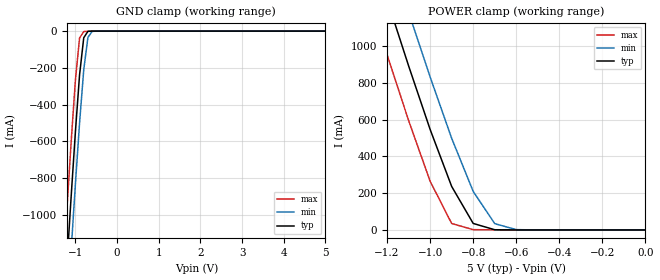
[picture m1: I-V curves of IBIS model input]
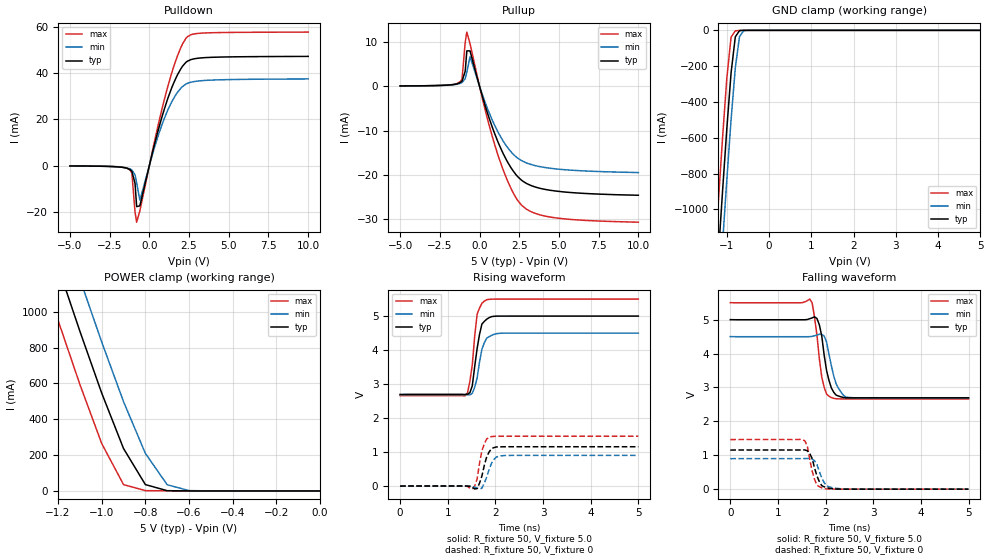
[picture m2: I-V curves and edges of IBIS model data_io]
| SOJ package &  Industrial operation.
[IBIS Ver]   3.2
[Comment Char]   |_char
[File name]   as7c1025b_soji.ibs
[File Rev]   1.0
[Date]   May 26, 2004 10:18:24 AM
[Source]
Alliance Semiconductor Corporation
[Notes]
This model  is for SOJ package & Industrial operation.
[Disclaimer]
Data is for modeling purpose only and is not guaranted.
This IBIS model is provided on an "AS IS" basis and Alliance Semiconductor makes
absolutely no warranty with respect to the information contained
herein.The entire risk as to quality and performance
is with the Customer. ACCORDINGLY, IN NO EVENT SHALL THE COMPANY BE
LIABLE FOR ANY DAMAGES, WHETHER IN CONTRACT OR TORT,INCLUDING ANY
LOST PROFITS OR OTHER INCIDENTAL, CONSEQUENTIAL, EXEMPLARY, OR
PUNITIVE DAMAGES ARISING OUT OF THE USE OR APPLICATION OF THE IBIS
model provided in this package.
[Copyright]
Alliance Semiconductor Corporation
| soj  Package & Industrial operation.
[Component]   AS7C1025B_SOJI
Si_location Pin
Timing_location Pin
[Manufacturer]   Alliance Semiconductor Corporation
[Package]
R_pkg   400.6m   286.6m   514.6m
L_pkg   8.541nH   5.418nH   11.663nH
C_pkg   1.870pF   1.203pF   2.538pF
[Pin] signal_name   model_name
1   A0   input
2   A1   input
3   A2   input
4   A3   input
5   NCE   input
6   IO0   data_io
7   IO1   data_io
8   VCC   POWER
9   GND   GND
10   IO2   data_io
11   IO3   data_io
12   NWE   input
13   A4   input
14   A5   input
15   A6   input
16   A7   input
17   A8   input
18   A9   input
19   A10   input
20   A11   input
21   A12   input
22   IO4   data_io
23   IO5   data_io
24   VCC   POWER
25   GND   GND
26   IO6   data_io
27   IO7   data_io
28   NOE   input
29   A13   input
30   A14   input
31   A15   input
32   A16   input
| Models and submodels in the file (2): input (Input), data_io (I/O)
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[Model]   input
Model_type Input
Vinh=2.2V
Vinl=0.8V
C_comp   4pF   4pF   4pF
[Model Spec]
[Temperature Range] 25   85   -40
[Voltage Range]   5.0   4.5   5.5
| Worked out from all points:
|   GND clamp passes 1 mA (typ) near -0.67 V on its own axis
|   POWER clamp passes 1 mA (typ) near -0.68 V on its own axis
[GND Clamp]
-5V       -16.01A    -16.28A    -15.75A
-1.3V     -1.622A    -1.916A    -1.322A
-1.2V     -1.253A    -1.547A    -953.4mA
-1.1V     -892.6mA   -1.184A    -596mA
-1V       -547.3mA   -832.1mA   -266.1mA
-900mV    -237.4mA   -499.3mA   -37.66mA
-800mV    -36.26mA   -209.9mA   -2.709mA
-700mV    -1.383mA   -34.75mA   -458.6uA
-600mV    -81.45uA   -1.835mA   -48.66uA
5V        292.5pA    86.47uA    -195.3pA
[POWER Clamp]
-5V       16.01A     16.27A     15.75A
-1.3V     1.621A     1.915A     1.322A
-1.2V     1.252A     1.546A     952.5mA
-1.1V     891.7mA    1.183A     594.7mA
-1V       546.1mA    831.3mA    264.7mA
-900mV    236.6mA    498.2mA    35.19mA
-800mV    35.4mA     209.4mA    1.73mA
-700mV    1.248mA    34.46mA    445.9uA
-600mV    85.03uA    1.813mA    86.82uA
0V        292.5pA    2.095nA    135pA
[Model]   data_io
Model_type I/O
Enable Active-High
Polarity Non-Inverting
Vinh=2.2V
Vinl=0.8V
Vref=1.728V
Vmeas=1.5V
Rref=168
Cref=30pF
C_comp   4pF   4pF   4pF
[Temperature Range] 25   85   -40
[Voltage Range]   5.0   4.5   5.5
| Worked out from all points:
|   slope of the pulldown table from 0 to 0.75 V, typ, clamps not added: 37.5 ohm
|   slope of the pullup table from 0 to 0.75 V, typ, clamps not added: 86.3 ohm
|   GND clamp passes 1 mA (typ) near -0.67 V on its own axis
|   POWER clamp passes 1 mA (typ) near -0.68 V on its own axis
|   falling waveform, R_fixture 50, V_fixture 5.0: 20-80 % time 166ps typ, 194ps min, 152ps max; typ from 5 V to 2.7 V
|   falling waveform, R_fixture 50, V_fixture 0: 20-80 % time 154ps typ, 156ps min, 138ps max; typ from 1.16 V to 0.002 V
|   rising waveform, R_fixture 50, V_fixture 5.0: 20-80 % time 146ps typ, 154ps min, 127ps max; typ from 2.69 V to 5 V
|   rising waveform, R_fixture 50, V_fixture 0: 20-80 % time 139ps typ, 149ps min, 124ps max; typ from 0 V to 1.16 V
[Pullup]
-5V       80uA       70uA       70uA
-1.2V     863uA      669uA      1.092mA
-1.1V     1.172mA    848uA      1.674mA
-900mV    3.44mA     1.737mA    9.973mA
-800mV    8.002mA    3.2mA      12.24mA
-600mV    8.001mA    6.666mA    9.641mA
300mV     -3.74mA    -3.123mA   -4.556mA
1.1V      -12.04mA   -9.899mA   -14.87mA
1.8V      -17.34mA   -14.01mA   -21.67mA
2.6V      -21.1mA    -16.71mA   -26.69mA
4.5V      -23.53mA   -18.55mA   -29.59mA
10V       -24.63mA   -19.51mA   -30.72mA
[Pulldown]
-5V       -150uA     -150uA     -120uA
-1.2V     -1.84mA    -1.479mA   -2.07mA
-1.1V     -2.529mA   -1.917mA   -3.263mA
-900mV    -7.724mA   -4.021mA   -20.18mA
-800mV    -17.8mA    -7.454mA   -24.55mA
-600mV    -17.46mA   -14.98mA   -19.72mA
300mV     8.509mA    7.287mA    9.717mA
1.1V      27.83mA    23.1mA     32.73mA
1.7V      38.37mA    31.04mA    46.23mA
2.3V      44.76mA    35.33mA    55.17mA
3.5V      46.82mA    36.93mA    57.52mA
10V       47.36mA    37.58mA    57.9mA
[GND Clamp]
-5V       -16.01A    -16.28A    -15.75A
-1.3V     -1.622A    -1.916A    -1.322A
-1.2V     -1.253A    -1.547A    -953.4mA
-1.1V     -892.6mA   -1.184A    -596mA
-1V       -547.3mA   -832.1mA   -266.1mA
-900mV    -237.4mA   -499.3mA   -37.66mA
-800mV    -36.26mA   -209.9mA   -2.709mA
-700mV    -1.383mA   -34.75mA   -458.6uA
-600mV    -81.45uA   -1.835mA   -48.66uA
5V        292.5pA    86.47uA    -195.3pA
[POWER Clamp]
-5V       16.01A     16.27A     15.75A
-1.3V     1.621A     1.915A     1.322A
-1.2V     1.252A     1.546A     952.5mA
-1.1V     891.7mA    1.183A     594.7mA
-1V       546.1mA    831.3mA    264.7mA
-900mV    236.6mA    498.2mA    35.19mA
-800mV    35.4mA     209.4mA    1.73mA
-700mV    1.248mA    34.46mA    445.9uA
-600mV    85.03uA    1.813mA    86.82uA
0V        292.5pA    2.095nA    135pA
[Falling Waveform]
R_fixture=50
V_fixture=5.0
V_fixture_min=4.5
V_fixture_max=5.5
0s        5V         4.5V       5.5V
1.667ns   5.026V     4.498V     5.606V
1.717ns   5.052V     4.506V     5.495V
1.768ns   5.082V     4.525V     5.07V
1.869ns   4.848V     4.57V      3.851V
1.97ns    3.957V     4.516V     3.009V
2.121ns   2.985V     3.641V     2.7V
2.222ns   2.773V     3.103V     2.667V
2.424ns   2.694V     2.719V     2.66V
5ns       2.696V     2.688V     2.66V
[Falling Waveform]
R_fixture=50
V_fixture=0
V_fixture_min=0
V_fixture_max=0
0s        1.155V     900.6mV    1.463V
1.566ns   1.159V     904.6mV    1.426V
1.616ns   1.134V     905.8mV    1.277V
1.667ns   1.055V     906.1mV    885.3mV
1.768ns   630.4mV    839.3mV    294mV
1.869ns   223.9mV    521.6mV    75.75mV
1.97ns    72.37mV    195.8mV    22.68mV
2.121ns   19.64mV    53.83mV    4.69mV
2.424ns   2.522mV    5.993mV    2.531mV
5ns       2.452mV    2.397mV    2.491mV
[Rising Waveform]
R_fixture=50
V_fixture=5.0
V_fixture_min=4.5
V_fixture_max=5.5
0s        2.694V     2.687V     2.658V
1.364ns   2.691V     2.687V     2.652V
1.414ns   2.701V     2.685V     2.741V
1.515ns   2.949V     2.729V     3.573V
1.566ns   3.52V      2.906V     4.421V
1.616ns   4.042V     3.178V     5.055V
1.717ns   4.764V     4.026V     5.372V
1.818ns   4.906V     4.348V     5.479V
2.121ns   4.996V     4.493V     5.496V
5ns       4.996V     4.497V     5.496V
[Rising Waveform]
R_fixture=50
V_fixture=0
V_fixture_min=0
V_fixture_max=0
0s        0V         647.5nV    0V
1.364ns   3.513mV    2.818mV    3.909mV
1.515ns   -32.3mV    -5.34mV    -77.13mV
1.616ns   -70.03mV   -59.72mV   206mV
1.717ns   298.9mV    -58.02mV   1.045V
1.818ns   866.3mV    269.8mV    1.389V
1.919ns   1.103V     673.6mV    1.458V
2.02ns    1.151V     855.7mV    1.464V
2.222ns   1.157V     901.3mV    1.465V
5ns       1.157V     902.9mV    1.466V
[Ramp]
R_load=50
dV/dt_r   6.942E-1/1.333E-10   5.418E-1/1.448E-10   8.793E-1/1.236E-10
dV/dt_f   1.383E+0/1.624E-10   1.087E+0/1.941E-10   1.704E+0/1.485E-10
|[End   data_io
